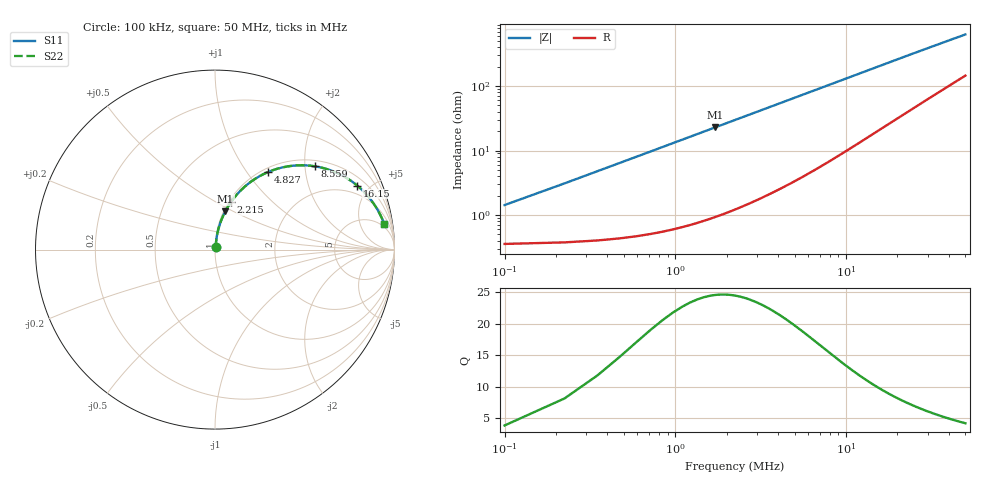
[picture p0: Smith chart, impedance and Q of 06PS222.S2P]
! Coilcraft 0603PS-222 Power Chip Inductor
! 19 February 2003
# MHZ S MA R 50
!Freq  MagS11  AngS11  MagS21  AngS21  MagS12  AngS12  MagS22  AngS22
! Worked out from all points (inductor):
!   403 points, 100 kHz to 50 MHz, reference 50 ohm
!   read as one part in series: L = 2.16 uH near 348.8 kHz
!   highest Q = 24.5 at 1.717 MHz (marker M1), where L = 2.12 uH
!   S11 on the Smith chart (normalised r, x): 100 kHz: 1.01, +0.03; 2.215 MHz: 1.02, +0.59; 4.827 MHz: 1.06, +1.27; 8.559 MHz: 1.15, +2.25; 16.15 MHz: 1.44, +4.20; 50 MHz: 4, +12
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0.1  0.01422 74.8  0.9964 -0.8  0.9964 -0.8  0.01422 74.8
0.2244  0.03081 81.3  0.9958 -1.8  0.9958 -1.8  0.03081 81.3
0.4732  0.06388 82.5  0.9937 -3.7  0.9937 -3.7  0.06388 82.5
0.5976  0.08026 82.1  0.9921 -4.6  0.9921 -4.6  0.08026 82.1
0.722  0.09653 81.5  0.9903 -5.5  0.9903 -5.5  0.09653 81.5
0.8464  0.1127 80.8  0.9882 -6.5  0.9882 -6.5  0.1127 80.8
1.0952  0.1445 79.2  0.9832 -8.3  0.9832 -8.3  0.1445 79.2
1.344  0.1758 77.5  0.9771 -10.1  0.9771 -10.1  0.1758 77.5
1.7172  0.2214 74.9  0.9662 -12.8  0.9662 -12.8  0.2214 74.9
2.2148  0.2796 71.4  0.9488 -16.2  0.9488 -16.2  0.2796 71.4
3.3344  0.3976 64.1  0.9003 -23.4  0.9003 -23.4  0.3976 64.1
4.8272  0.5257 55.5  0.8249 -31.7  0.8249 -31.7  0.5257 55.5
6.4444  0.6297 47.8  0.7416 -38.9  0.7416 -38.9  0.6297 47.8
8.4348  0.7192 40.3  0.6483 -45.9  0.6483 -45.9  0.7192 40.3
8.5592  0.7237 39.9  0.643 -46.2  0.643 -46.2  0.7237 39.9
11.918  0.812 31.2  0.5194 -54.0  0.5194 -54.0  0.812 31.2
16.1476  0.8694 24.2  0.4119 -59.8  0.4119 -59.8  0.8694 24.2
16.7696  0.8751 23.4  0.3995 -60.5  0.3995 -60.5  0.8751 23.4
25.1044  0.9199 16.3  0.2827 -65.6  0.2827 -65.6  0.9199 16.3
33.4392  0.9386 12.4  0.2184 -67.6  0.2184 -67.6  0.9386 12.4
41.774  0.9485 10.0  0.1781 -68.2  0.1781 -68.2  0.9485 10.0
50  0.9544 8.5  0.151 -68.3  0.151 -68.3  0.9544 8.5
